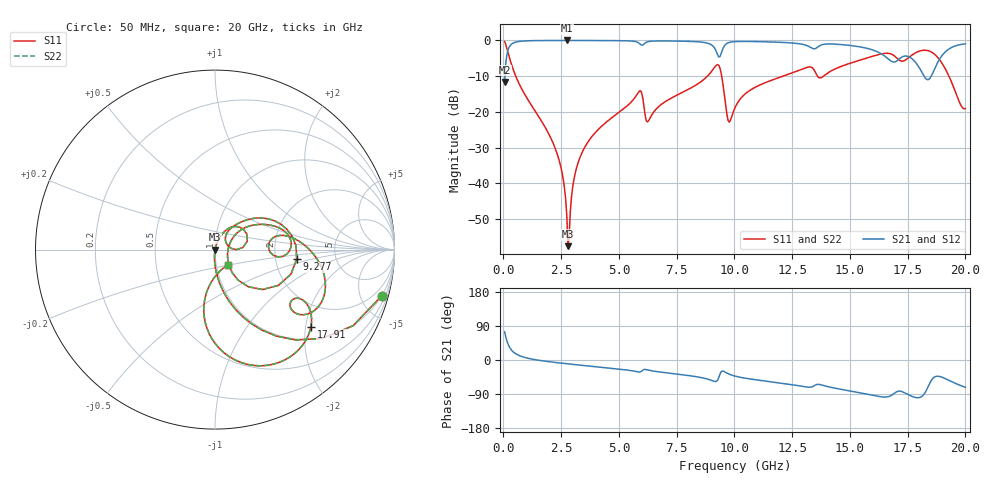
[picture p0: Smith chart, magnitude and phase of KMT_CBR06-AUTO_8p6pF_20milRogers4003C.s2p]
! Data measured by Modelithics Inc. support@modelithics.com 813-866-6335
! KEMET CBR06-AUTO 8.6pF, Pad Width= 0.851mm, Pad Length= 0.64mm, Pad Gap= 0.62mm, 20mil Rogers 4003C substrate Data, January 2022
# hz S ma R 50
! 2 Port Network Data from SP1.SP block
! freq  magS11  angS11  magS21  angS21  magS12  angS12  magS22  angS22
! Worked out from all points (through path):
!   401 points, 50 MHz to 20 GHz, reference 50 ohm
!   highest |S21| = -0.01 dB at 2.743 GHz (marker M1); lowest = -11.6 dB at 50 MHz (marker M2)
!   group delay of S21, straight-line fit = 13.7 ps
!   lowest |S11| = -57.6 dB at 2.793 GHz (marker M3), VSWR 1.00, Z = 50.1 - j0.111 ohm
!   |S11| at or under -10 dB: 532.4 MHz to 8.833 GHz (8.3 GHz wide, 177 % of centre); 9.447 GHz to 12.11 GHz (2.658 GHz wide, 24.7 % of centre); 19.29 GHz to end of sweep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
!   |S22| runs from -57.6 to -0.3 dB; largest |S21 - S12| = 0
!   S11 on the Smith chart (normalised r, x): 50 MHz: 0.98, -7.26; 9.277 GHz: 2.63, -0.36; 17.91 GHz: 1.31, -2.14; 20 GHz: 1.14, -0.19
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5e7  0.9648 -15.4  0.2626 74.6  0.2626 74.6  0.9648 -15.4
2.99375e8  0.5187 -59.8  0.8543 30.1  0.8543 30.1  0.5187 -59.8
5.98625e8  0.2816 -75.7  0.9589 14.2  0.9589 14.2  0.2816 -75.7
2.2445e9  0.03061 -95.0  0.9986 -6.5  0.9986 -6.5  0.03061 -95.0
2.54375e9  0.01369 -94.9  0.999 -8.6  0.999 -8.6  0.01369 -94.9
2.74325e9  0.003537 -85.3  0.999 -9.9  0.999 -9.9  0.003537 -85.3
2.793125e9  0.001317 -57.2  0.999 -10.2  0.999 -10.2  0.001317 -57.2
3.391625e9  0.02644 73.9  0.9985 -13.9  0.9985 -13.9  0.02644 73.9
5.8355e9  0.1855 42.4  0.9326 -31.6  0.9326 -31.6  0.1855 42.4
6.2345e9  0.07216 28.4  0.9561 -26.1  0.9561 -26.1  0.07216 28.4
6.73325e9  0.1195 54.5  0.9839 -31.4  0.9839 -31.4  0.1195 54.5
8.877875e9  0.3275 32.2  0.9071 -51.1  0.9071 -51.1  0.3275 32.2
9.276875e9  0.4583 -6.8  0.6252 -52.8  0.6252 -52.8  0.4583 -6.8
9.72575e9  0.07589 -23.4  0.9255 -36.1  0.9255 -36.1  0.07589 -23.4
1.0025e10  0.1142 32.3  0.9635 -42.5  0.9635 -42.5  0.1142 32.3
1.336662e10  0.4148 -1.0  0.776 -70.5  0.776 -70.5  0.4148 -1.0
1.511225e10  0.4911 3.7  0.8419 -82.9  0.8419 -82.9  0.4911 3.7
1.670825e10  0.6566 -29.4  0.5353 -95.8  0.5353 -95.8  0.6566 -29.4
1.790525e10  0.6864 -38.9  0.4638 -99.5  0.4638 -99.5  0.6864 -38.9
1.86035e10  0.6645 -74.2  0.3597 -47.7  0.3597 -47.7  0.6645 -74.2
1.915212e10  0.3874 -98.7  0.7013 -49.8  0.7013 -49.8  0.3874 -98.7
2e10  0.1109 -49.5  0.8959 -71.9  0.8959 -71.9  0.1109 -49.5
